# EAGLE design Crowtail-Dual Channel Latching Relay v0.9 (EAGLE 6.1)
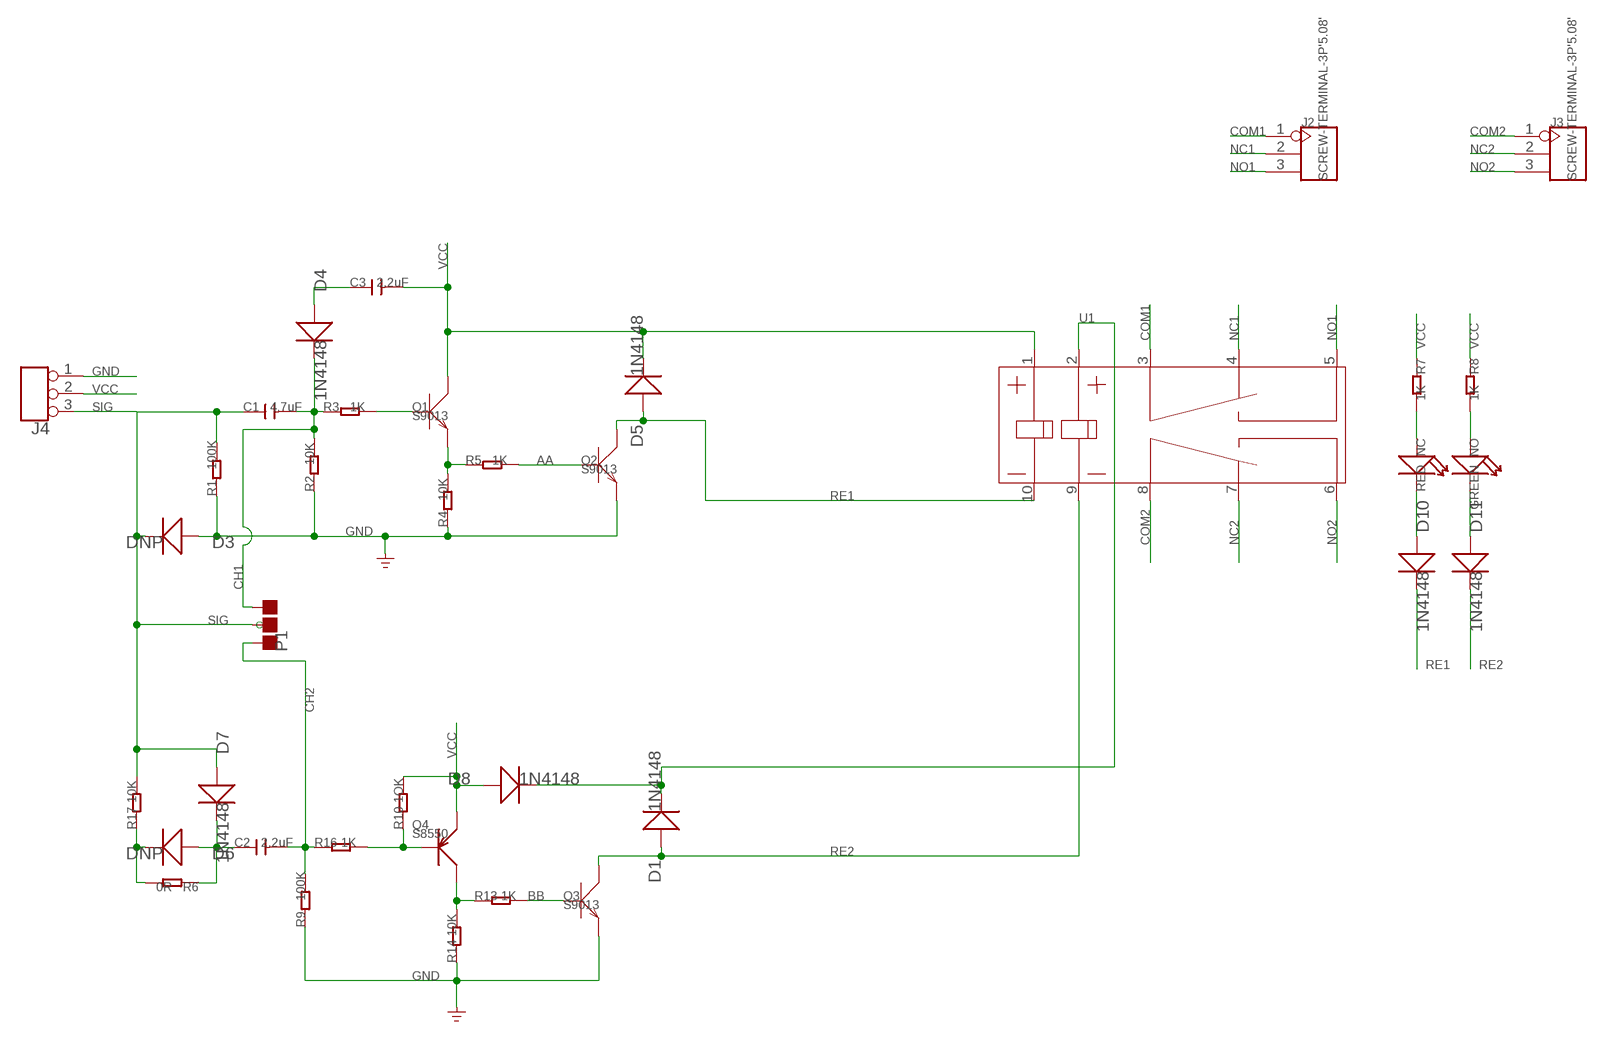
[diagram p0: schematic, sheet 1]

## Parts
C1  4.7uF  C-0805  [C0805]
C2  2.2uF  C-0805  [C0805]
C3  2.2uF  C-0805  [C0805]
D1  1N4148  D'1N4148-SMD'  [DO-35-SMD]
D3  DNP  D'1N4148-SMD'  [DO-35-SMD]
D4  1N4148  D'1N4148-SMD'  [DO-35-SMD]
D5  1N4148  D'1N4148-SMD'  [DO-35-SMD]
D6  DNP  D'1N4148-SMD'  [DO-35-SMD]
D7  1N4148  D'1N4148-SMD'  [DO-35-SMD]
D8  1N4148  D'1N4148-SMD'  [DO-35-SMD]
D10  1N4148  D'1N4148-SMD'  [DO-35-SMD]
D11  1N4148  D'1N4148-SMD'  [DO-35-SMD]
J2  SCREW-TERMINAL-3P'5.08'  [3P-5.08]
J3  SCREW-TERMINAL-3P'5.08'  [3P-5.08]
J4  TINKER_3P_DIP  [3P_2.0_DIP]
NC  RED  LED'0603'  [LED-0603]
NO  GREEN  LED'0603'  [LED-0603]
P1  PAD-JUMPER-3P-40*40  [3P-SMD-4.1X1.5]
Q1  S9013  TRANSISTOR-NPN-SOT23  [SOT23]
Q2  S9013  TRANSISTOR-NPN-SOT23  [SOT23]
Q3  S9013  TRANSISTOR-NPN-SOT23  [SOT23]
Q4  S8550  TRANSISTOR-PNP-SOT23  [SOT23]
R1  100K  R-0603  [R0603]
R2  10K  R-0603  [R0603]
R3  1K  R-0603  [R0603]
R4  10K  R-0603  [R0603]
R5  1K  R-0603  [R0603]
R6  0R  R-0603  [R0603]
R7  1K  R-0603  [R0603]
R8  1K  R-0603  [R0603]
R9  100K  R-0603  [R0603]
R10  1OK  R-0603  [R0603]
R13  1K  R-0603  [R0603]
R14  10K  R-0603  [R0603]
R16  1K  R-0603  [R0603]
R17  10K  R-0603  [R0603]
U1  RELAY-HFD2/005-S-L2'HFD2/005-S-L2'  [10P-20.2X10.2X10.6]

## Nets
AA: Q2.1(B) R5.2
BB: Q3.1(B) R13.2
CH1: C1.2 D4.C(-) P1.00(L) R2.2 R3.1
CH2: C2.2 P1.11(R) R9.2 R16.1
COM1: J2.1 U1.3
COM2: J3.1 U1.8
GND: D3.A(+) J4.1 Q2.2(E) Q3.2(E) R1.1 R2.1 R4.1 R9.1 R14.1
N$1: NO.+ R8.2
N$3: C3.1 D4.A(+)
N$4: Q1.1(B) R3.2
N$5: Q1.2(E) R4.2 R5.1
N$6: D10.A(+) NC.-
N$7: D11.A(+) NO.-
N$9: NC.+ R7.2
N$11: D6.C(-) R6.2 R17.1
N$12: C2.1 D6.A(+) D7.C(-) R6.1
N$15: Q4.1(B) R10.1 R16.2
N$17: D1.C(-) D8.C(-) U1.2
N$21: Q4.3(C) R13.1 R14.2
NC1: J2.2 U1.4
NC2: J3.2 U1.7
NO1: J2.3 U1.5
NO2: J3.3 U1.6
RE1: D5.A(+) D10.C(-) Q2.3(C) U1.10
RE2: D1.A(+) D11.C(-) Q3.3(C) U1.9
SIG: C1.1 D3.C(-) D7.A(+) J4.3 P1.MM(C) R1.2 R17.2
VCC: C3.2 D5.C(-) D8.A(+) J4.2 Q1.3(C) Q4.2(E) R7.1 R8.1 R10.2 U1.1

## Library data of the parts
C1-C3 = Discrete:C*: Ceramic Capacitors
D1 D3-D8 D10 D11 = Discrete:D*
J2 J3 = Connector:SCREW-TERMINAL-3P
J4 = Connector:TINKER_3P_DIP
NC NO = Discrete:LED*
P1 = Discrete:PAD-JUMPER-3P; PARTNO: DNP
Q1-Q3 = Discrete:TRANSISTOR-NPN*: NPN audion
Q4 = Discrete:TRANSISTOR-PNP*: PNP audion
R1-R10 R13 R14 R16 R17 = Discrete:R*
U1 = template:RELAY-HFD2/005-S-L2: 2 coils latching

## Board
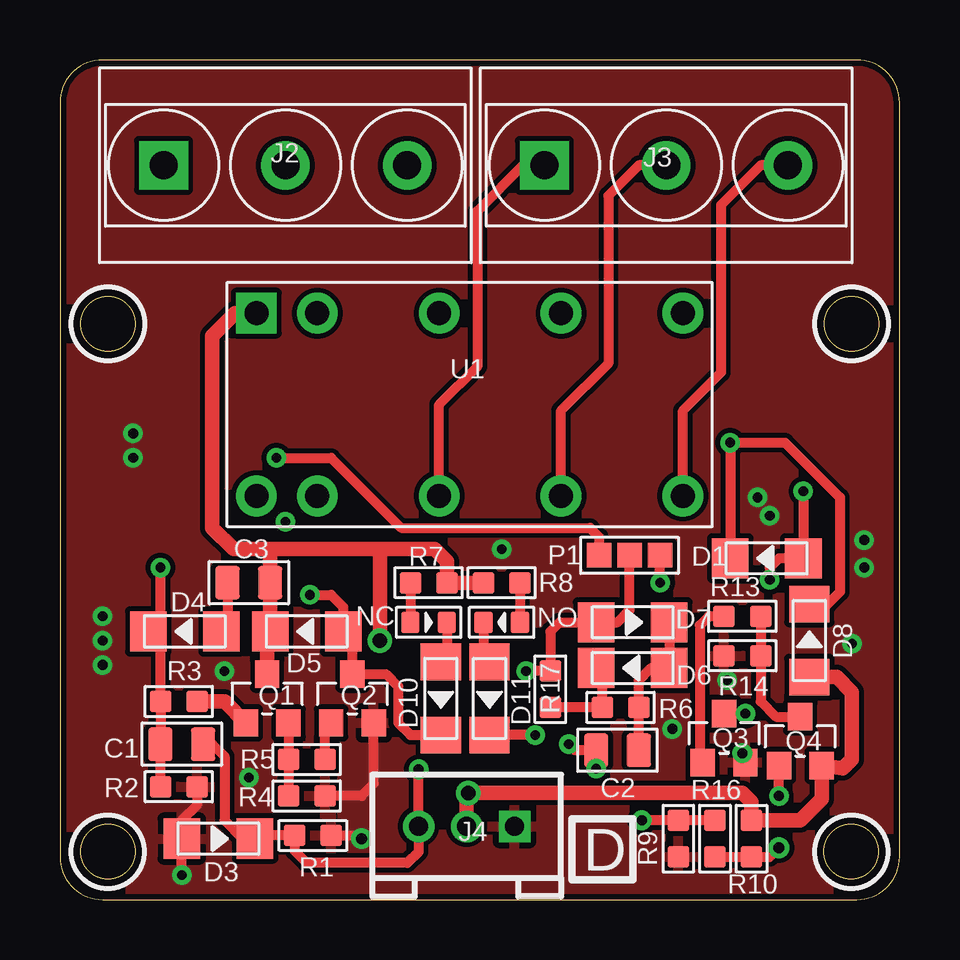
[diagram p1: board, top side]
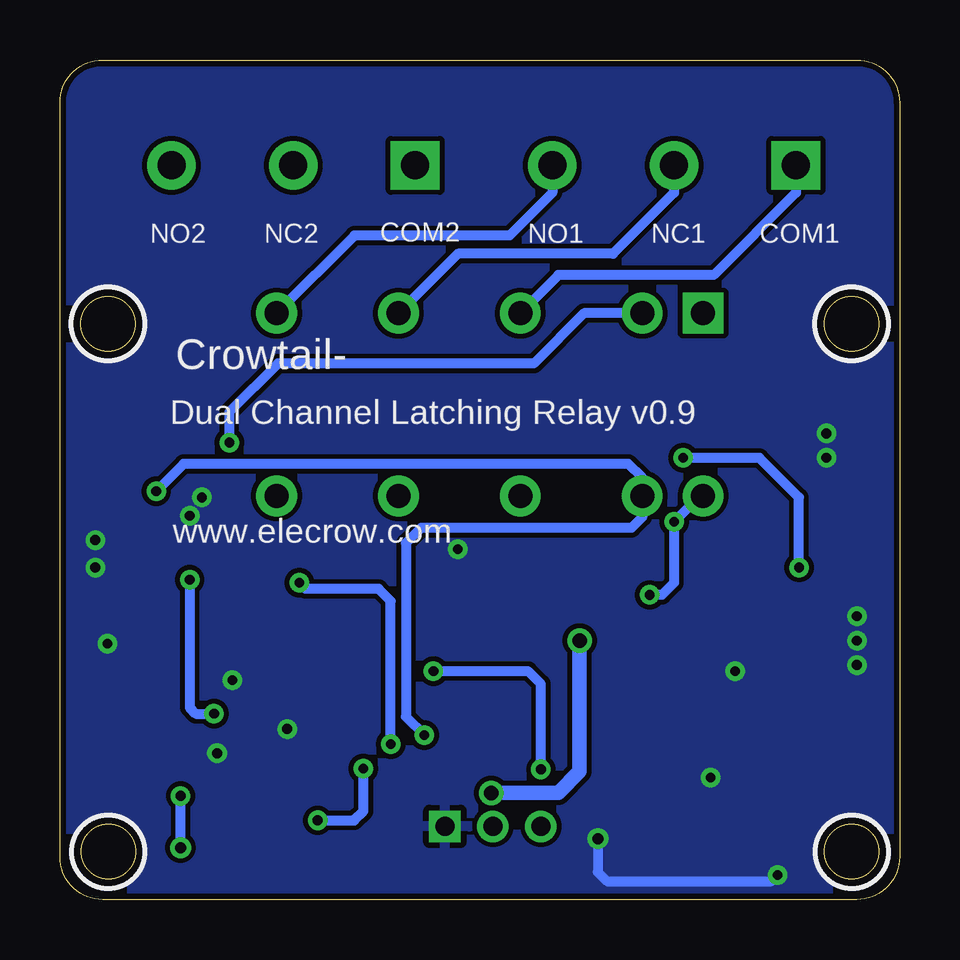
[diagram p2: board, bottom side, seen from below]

Size 35 x 35 mm. Coordinates in mm from the lower left corner, seen from the top.
Outline: 1.78,0 33.22,0 arc90 35,1.78 35,33.22 arc90 33.22,35 1.78,35 arc90 0,33.22 0,1.78 arc90 1.78,0
Outline: circle at 33,24 radius 1.14
Outline: circle at 2,2 radius 1.14
Outline: circle at 32.99,2 radius 1.14
Outline: circle at 2,24 radius 1.14
Copper layers (1*16): Top 0.035mm / dielectric 1.5mm / Bottom 0.035mm
Design rules: minimum track width 10mil, minimum drill 12mil, track to track 8mil, track to pad 8mil, pad to pad 8mil, via to via 8mil, smd to smd 0mil, copper to edge 10mil, drill to drill 8mil, minimum pad ring 10mil, minimum via ring 8mil, stop-mask expansion 4mil, vias tented up to drill 100mil, thermal gap 10mil
tRestrict: area 31.5,22.5 to 34.5,25.5; area 0.5,0.5 to 3.5,3.5; area 31.5,0.5 to 34.5,3.5; area 0.5,22.5 to 3.5,25.5
bRestrict: area 31.5,22.5 to 34.5,25.5; area 0.5,0.5 to 3.5,3.5; area 31.5,0.5 to 34.5,3.5; area 0.5,22.5 to 3.5,25.5

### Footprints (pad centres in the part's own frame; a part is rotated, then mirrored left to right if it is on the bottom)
C0805 = smd 1.016 x 1.397: 1 -0.889,0; 2 0.889,0
DO-35-SMD = smd 1.524 x 1.676: A -1.524,0; C 1.524,0
3P-5.08 = drill 1.168 pad 2.032 square: 1 0,5.08 | drill 1.168 pad 2.032: 2 0,0; 3 0,-5.08
3P_2.0_DIP = drill 0.8 pad 1.27 square: 1 -2,0 | drill 0.8 pad 1.27: 2 0,0; 3 2,0
LED-0603 = smd 0.762 x 0.889: + -0.762,0; - 0.762,0
3P-SMD-4.1X1.5 = smd 1.016 x 1.016: 00 -1.27,0; 11 1.27,0; MM 0,0
SOT23 = smd 1.016 x 1.143: 1 -0.889,-1.016; 2 0.889,-1.016; 3 0,1.016
R0603 = smd 0.889 x 0.889: 1 -0.762,0; 2 0.762,0
10P-20.2X10.2X10.6 = drill 1 pad 1.7 square: 1 -8.89,3.81 | drill 1 pad 1.7: 2 -6.35,3.81; 3 -1.27,3.81; 4 3.81,3.81; 5 8.89,3.81; 6 8.89,-3.81; 7 3.81,-3.81; 8 -1.27,-3.81; 9 -6.35,-3.81; 10 -8.89,-3.81

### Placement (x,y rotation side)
C1  5.08,6.48 180 top
C2  23.24,6.22 180 top
C3  7.87,13.21 0 top
D1  29.46,14.22 180 top
D3  6.6,2.54 0 top
D4  5.21,11.18 180 top
D5  10.29,11.18 180 top
D6  23.88,9.65 180 top
D7  23.88,11.56 0 top
D8  31.24,10.79 90 top
D10  15.88,8.38 270 top
D11  17.91,8.38 270 top
J2  9.4,30.61 90 top
J3  25.27,30.61 90 top
J4  16.95,3.05 180 top
NC  15.37,11.56 0 top
NO  18.41,11.56 180 top
P1  23.75,14.35 0 top
Q1  8.64,8.38 0 top
Q2  12.19,8.38 0 top
Q3  27.69,6.73 0 top
Q4  30.86,6.6 0 top
R1  10.54,2.67 180 top
R2  4.95,4.7 180 top
R3  4.95,8.26 0 top
R4  10.29,4.32 180 top
R5  10.29,5.84 0 top
R6  23.37,8 180 top
R7  15.37,13.21 180 top
R8  18.41,13.21 0 top
R9  25.78,2.54 90 top
R10  28.83,2.54 90 top
R13  28.45,11.81 180 top
R14  28.45,10.16 0 top
R16  27.3,2.54 270 top
R17  20.45,8.76 90 top
U1  17.08,20.64 0 top

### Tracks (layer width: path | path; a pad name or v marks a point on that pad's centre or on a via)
AA
  Top 0.406: R5.2 11.05,7.11 Q2.1
BB
  Top 0.406: R13.2 27.05,11.81 26.67,11.43 26.67,5.84 Q3.1
CH1  (via drill 0.41)
  Top 0.406: R2.2 C1.2 R3.1 4.19,10.67 | 4.19,10.67 D4.C | 4.19,10.67 v4.19,13.84 | v9.02,18.41 11.3,18.41 14.22,15.49 22.1,15.49 22.48,15.11 P1.00
  Bottom 0.406: v4.19,13.84 4.19,16.76 5.84,18.41 v9.02,18.41
CH2  (via drill 0.41)
  Top 0.406: R16.1 R9.2 v24.26,3.3 | v22.35,5.46 C2.2 21.46,6.22 v21.21,6.48 | v25.02,13.21 P1.11
  Bottom 0.406: v24.26,3.3 22.73,3.3 22.35,3.68 v22.35,5.46 | v21.21,6.48 21.21,12.45 21.72,12.95 24.77,12.95 v25.02,13.21
COM1
  Bottom 0.406: J2.1 4.32,29.46 7.75,26.04 14.22,26.04 U1.3
COM2
  Top 0.406: J3.1 19.3,30.61 17.4,28.7 17.4,22.23 15.81,20.64 U1.8
GND  (via drill 0.41, 0.46)
  Top 0.406: Q2.2 13.08,4.83 12.57,4.32 R4.1 | R1.1 12.45,2.67 v12.57,2.54 | v5.08,1.02 D3.A 5.08,3.3 5.71,3.94 R2.1
  Bottom 0.406: v12.57,2.54 12.57,1.14 12.19,0.76 5.33,0.76 v5.08,1.02
  other vias: 27.81,9.14 28.45,6.1 33.02,10.67 25.53,7.11 18.41,14.61 1.78,11.81 1.78,10.79 1.78,9.78 6.86,9.53 7.87,5.08 29.08,16.76 29.59,16 33.53,13.84 33.53,14.99 3.05,19.43 3.05,18.41
  pour Top: 33.53,-0.25 1.52,-0.25 arc-90 -0.25,1.52 -0.25,33.53 arc-90 1.52,35.31 33.53,35.31 arc-90 35.31,33.53 35.31,1.52 arc-90
  pour Bottom: 35.31,33.53 35.31,1.52 arc-90 33.53,-0.25 1.52,-0.25 arc-90 -0.25,1.52 -0.25,33.53 arc-90 1.52,35.31 33.53,35.31 arc-90
N$1
  Top 0.406: R8.2 NO.+
N$3
  Top 0.406: C3.1 6.99,11.43 D4.A
N$4
  Top 0.61: R3.2 6.86,8.26 Q1.1
N$5
  Top 0.406: Q1.2 R5.1 R4.2
N$6
  Top 0.406: NC.- 16.13,10.16 D10.A
N$7
  Top 0.406: NO.- 17.65,10.16 D11.A
N$9
  Top 0.406: R7.2 NC.+
N$11
  Top 0.406: 22.61,9.78 D6.C 22.61,9.53 R6.2 R17.1
N$12
  Top 0.406: C2.1 R6.1 24.13,9.14 24.64,9.65 D6.A D7.C
N$15  (via drill 0.41, 0.46)
  Top 0.406: R16.2 R10.1 29.59,1.78 v29.97,2.16 | v29.97,4.32 Q4.1
  Bottom 0.406: v29.97,2.16 v29.97,4.32
N$17  (via drill 0.41)
  Top 0.406: D1.C v27.94,19.05 30.23,19.05 32.51,16.76 32.51,12.83 32,12.32 D8.C
  Bottom 0.406: U1.2 13.15,24.45 15.24,22.35 25.91,22.35 27.94,20.32 v27.94,19.05
N$21
  Top 0.406: R13.1 R14.2 29.21,8.26 29.84,7.62 Q4.3
NC1
  Bottom 0.406: J2.2 9.4,29.46 11.94,26.92 18.41,26.92 U1.4
NC2
  Top 0.406: J3.2 24.13,30.61 22.86,29.34 22.86,22.35 20.89,20.38 U1.7
NO1
  Bottom 0.406: J2.3 14.48,29.46 16.26,27.69 22.73,27.69 U1.5
NO2
  Top 0.406: J3.3 29.21,30.61 27.56,28.96 27.56,21.97 25.97,20.38 U1.6
RE1  (via drill 0.41)
  Top 0.406: v10.41,12.7 11.3,12.7 11.81,12.19 D5.A 12.19,10.79 Q2.3 13.59,9.4 14.1,8.89 14.1,7.37 14.61,6.86 15.75,6.86 15.88,6.73 D10.C
  Bottom 0.406: v10.41,12.7 9.91,12.7 9.4,13.21 v9.4,15.75 8.32,16.82 U1.10
RE2  (via drill 0.41)
  Top 0.406: v29.59,13.34 29.59,13.84 29.97,14.22 D1.A | v28.57,7.75 Q3.3 | 30.99,14.1 D1.A | v30.99,17.02 D1.A | v19.81,6.86 D11.C
  Bottom 0.406: v29.59,13.34 29.59,8 29.34,7.75 v28.57,7.75 | v30.99,17.02 29.84,18.16 11.3,18.16 10.73,17.59 U1.9 10.73,15.94 11.18,15.49 19.94,15.49 20.57,14.86 20.57,7.62 v19.81,6.86
SIG  (via drill 0.41)
  Top 0.406: v14.95,5.43 J4.3 14.95,2 14.48,1.52 10.29,1.52 9.78,2.03 R1.2 8.26,2.67 D3.C 7.62,2.54 6.86,3.3 6.86,5.97 6.35,6.48 C1.1 | v19.43,9.53 R17.2 20.45,11.18 20.83,11.56 D7.A 23.24,11.56 23.75,12.06 P1.MM
  Bottom 0.406: v19.43,9.53 15.49,9.53 14.95,8.98 v14.95,5.43
VCC  (via drill 0.61)
  Top 0.61: 13.34,14.61 15.62,14.61 16.13,14.1 R7.1 R8.1 | 13.34,14.61 v13.34,10.79 | J4.2 16.95,4.38 v17.02,4.45 28.45,4.45 28.83,4.06 R10.2 30.86,3.3 31.75,4.19 Q4.2 32.64,5.46 33.02,5.84 33.02,8.64 32.38,9.27 D8.A | 8.76,14.61 7.24,14.61 6.35,15.49 6.35,23.5 7.3,24.45 U1.1 | 8.76,14.61 13.34,14.61 | 8.76,14.61 C3.2 D5.C 8.64,11.05 Q1.3
  Bottom 0.61: v13.34,10.79 13.34,5.33 14.22,4.45 v17.02,4.45

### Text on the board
tPlace: D
bPlace: COM1 | NC1 | NO1 | NC2 | NO2 | COM2 | Crowtail- | Dual Channel Latching Relay v0.9 | www.elecrow.com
